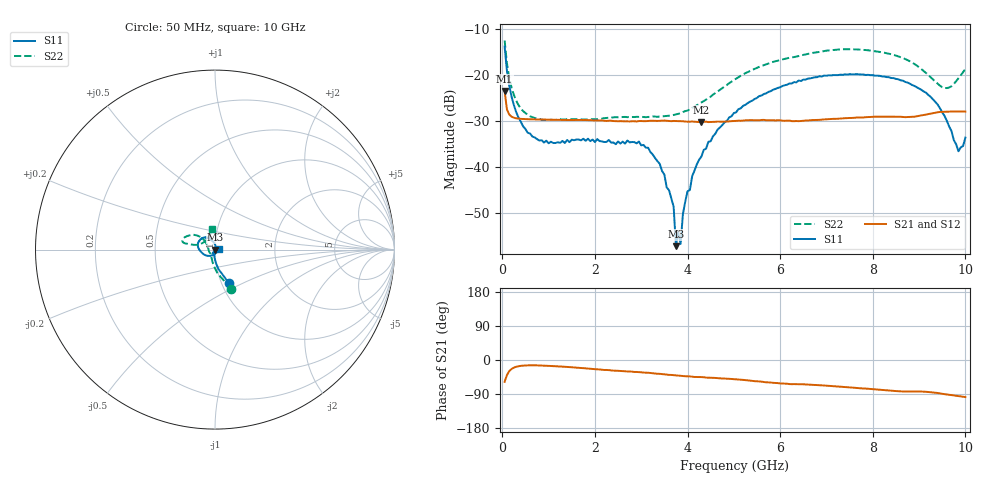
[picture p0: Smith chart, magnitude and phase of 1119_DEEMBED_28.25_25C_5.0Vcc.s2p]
!Hittite Microwave Corp.
!Digital Attenuator/PhaseShifter Rev 1.4.0
!Filename: C:\DATA\DATA\1119_DEEMBED_28.25_25C_5.0Vcc.s2p
!VNA ID: Agilent Technologies,N5224A,MY51441122,A.10.45.03
!Device type:
!2 Port Calibration.
!Temp(C): 25
!Lot Number:
!Serial Number:
!Operator:
!Misc:
!Attenuator:  28.250
# GHZ S DB R 50.0
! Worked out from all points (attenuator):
!   200 points, 50 MHz to 10 GHz, reference 50 ohm
!   highest |S21| = -23.50 dB at 50 MHz (marker M1); lowest = -30.2 dB at 4.3 GHz (marker M2)
!   lowest |S11| = -57.1 dB at 3.75 GHz (marker M3), VSWR 1.00, Z = 50.1 - j0.126 ohm
!   |S11| at or under -10 dB: start of sweep to end of sweep
!   |S22| runs from -29.8 to -12.6 dB; largest |S21 - S12| = 0.00012
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0.05  -13.88 -67.4  -23.50 -57.6  -23.51 -57.6  -12.56 -67.5
0.1  -19.10 -79.8  -27.50 -39.9  -27.50 -39.8  -17.51 -84.0
0.2  -24.73 -89.5  -29.07 -23.7  -29.08 -23.8  -22.78 -100.6
0.55  -32.57 -104.7  -29.63 -14.1  -29.64 -14.2  -28.65 -126.4
1  -34.84 -114.5  -29.74 -15.5  -29.73 -15.5  -29.73 -137.3
1.75  -33.86 -119.9  -29.81 -21.6  -29.81 -21.7  -29.67 -140.9
2.95  -34.47 -101.6  -30.02 -31.9  -30.03 -31.9  -29.13 -160.2
3.4  -39.30 -99.1  -29.98 -36.5  -29.98 -36.5  -29.05 -173.7
3.7  -48.58 -74.1  -30.00 -40.0  -30.01 -40.1  -28.70 175.1
3.75  -57.14 -64.6  -30.01 -40.7  -30.01 -40.8  -28.57 173.1
3.8  -54.09 -28.0  -30.04 -41.3  -30.05 -41.4  -28.46 170.3
3.85  -56.65 37.4  -30.06 -41.7  -30.07 -41.8  -28.30 168.3
3.9  -50.22 45.7  -30.07 -42.3  -30.08 -42.4  -28.09 166.5
4  -45.24 57.3  -30.16 -43.1  -30.17 -43.2  -27.76 161.8
4.3  -37.72 78.5  -30.25 -45.1  -30.26 -45.2  -25.99 150.4
5.05  -28.12 98.5  -29.99 -51.0  -30.01 -51.0  -20.83 138.6
6.7  -20.65 135.1  -29.81 -65.6  -29.82 -65.6  -15.26 153.8
8.35  -20.52 173.1  -29.09 -80.6  -29.08 -80.6  -15.43 168.1
9.15  -23.87 -151.7  -28.62 -83.8  -28.63 -83.9  -19.61 165.4
9.55  -28.92 -116.0  -28.00 -90.1  -28.01 -90.2  -22.86 138.0
9.85  -36.57 -41.6  -27.94 -95.1  -27.95 -95.1  -20.76 105.8
10  -33.62 14.7  -27.98 -97.8  -27.98 -97.8  -18.73 98.2
